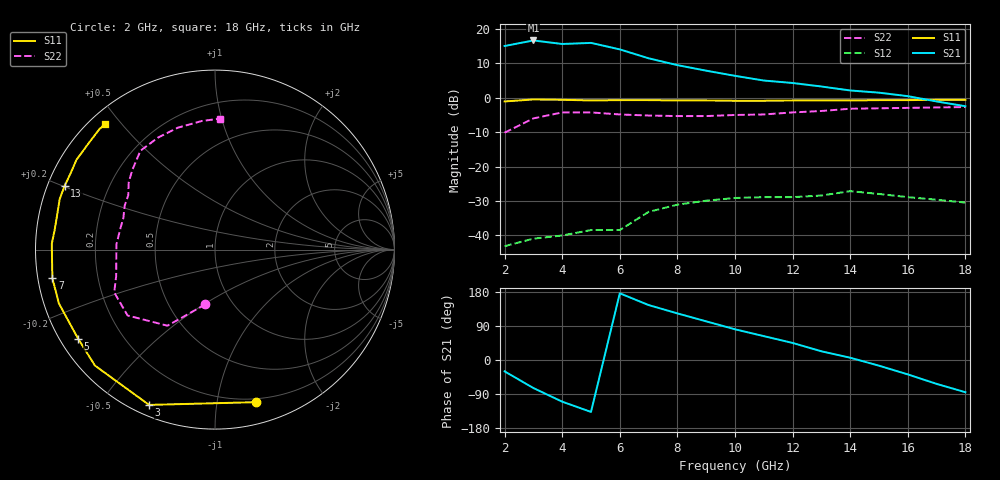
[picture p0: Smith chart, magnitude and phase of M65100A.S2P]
!  MGA-65100 S PARAMETERS: smoothed data
!  Vds=10V  Id=158mA  LAST UPDATED 07-22-92
# ghz s ma r 50
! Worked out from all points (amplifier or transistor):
!   17 points, 2 GHz to 18 GHz, reference 50 ohm
!   highest |S21| = 16.6 dB at 3 GHz (marker M1)
!   |S21| within 3 dB of that: start of sweep to 6.159 GHz
!   unconditionally stable (mu >= 1): start of sweep to 2.802 GHz; 3.588 GHz to end of sweep
!   at 4 GHz: K = 1.14, MAG = 25.5 dB, |S12| = -40.0 dB
!   at 10 GHz: K = 1.44, MAG = 13.8 dB, |S12| = -29.1 dB
!   at 18 GHz: K = 1.25, MAG = 11.0 dB, |S12| = -30.5 dB
!   S11 on the Smith chart (normalised r, x): 2 GHz: 0.17, -1.29; 3 GHz: 0.04, -0.66; 5 GHz: 0.05, -0.30; 7 GHz: 0.04, -0.09; 13 GHz: 0.05, +0.20; 18 GHz: 0.04, +0.46
2  0.88 -75.0  5.61 -30.0  0.007 131.0  0.31 -100.0
3  0.94 -113.0  6.75 -74.0  0.009 118.0  0.5 -122.0
4  0.93 -136.0  6 -110.0  0.01 55.0  0.61 -143.0
5  0.91 -147.0  6.22 -137.0  0.012 -5.0  0.61 -157.0
6  0.92 -161.0  5.01 176.0  0.012 53.0  0.57 -165.0
7  0.92 -170.0  3.72 145.0  0.022 74.0  0.55 177.0
8  0.91 -176.0  2.96 123.0  0.028 73.0  0.54 167.0
9  0.91 178.0  2.46 102.0  0.032 70.0  0.54 161.0
10  0.9 173.0  2.07 81.0  0.035 68.0  0.56 154.0
11  0.9 168.0  1.77 63.0  0.036 65.0  0.57 148.0
12  0.91 162.0  1.63 45.0  0.036 63.0  0.61 142.0
13  0.91 157.0  1.45 23.0  0.038 61.0  0.64 136.0
14  0.91 152.0  1.27 6.0  0.044 58.0  0.69 127.0
15  0.92 147.0  1.18 -15.0  0.04 44.0  0.7 117.0
16  0.92 140.0  1.05 -38.0  0.036 38.0  0.71 107.0
17  0.93 134.0  0.88 -63.0  0.033 30.0  0.72 96.0
18  0.93 131.0  0.75 -85.0  0.03 20.0  0.73 88.0
